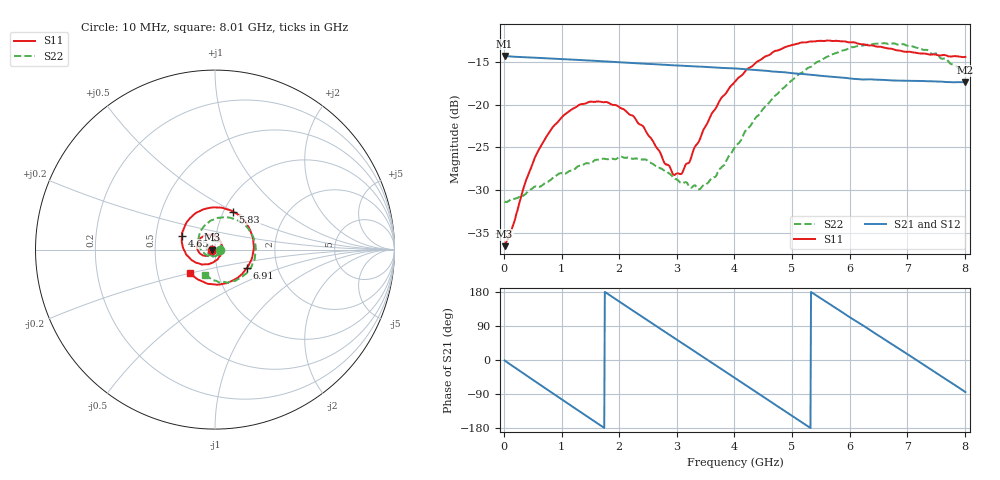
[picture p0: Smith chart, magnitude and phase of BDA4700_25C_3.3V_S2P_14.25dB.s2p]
!Agilent Technologies,E5071B,MY42404982,A.09.10
!Date: Mon Oct 20 18:09:01 2025
!Data & Calibration Information:
!Freq	S11:SOLT2(ON)	S21:SOLT2(ON)	S12:SOLT2(ON)	S22:SOLT2(ON)
# Hz S RI R 50
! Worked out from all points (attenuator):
!   801 points, 10 MHz to 8.01 GHz, reference 50 ohm
!   highest |S21| = -14.34 dB at 10 MHz (marker M1); lowest = -17.4 dB at 8 GHz (marker M2)
!   lowest |S11| = -36.5 dB at 10 MHz (marker M3), VSWR 1.03, Z = 48.5 - j0.125 ohm
!   |S11| at or under -10 dB: start of sweep to end of sweep
!   |S22| runs from -31.4 to -12.8 dB; largest |S21 - S12| = 0.0022
!   S11 on the Smith chart (normalised r, x): 10 MHz: 0.97, -0.00; 4.65 GHz: 0.68, +0.11; 5.83 GHz: 1.11, +0.50; 6.91 GHz: 1.39, -0.30; 8.01 GHz: 0.73, -0.19
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1e7  -0.0149 -0.00129  0.1917 -0.00424  0.1917 -0.00433  0.0271 -0.00099
6e8  -0.0417 -0.0347  0.0863 -0.166  0.0861 -0.166  0.0118 -0.031
1.01e9  -0.0815 -0.0238  -0.0467 -0.1781  -0.0466 -0.1781  -0.0196 -0.0347
1.35e9  -0.1002 0.0105  -0.1381 -0.1179  -0.1381 -0.1181  -0.0417 -0.0142
1.71e9  -0.087 0.0555  -0.1784 -0.012  -0.1785 -0.0118  -0.045 0.0174
2.07e9  -0.0458 0.0819  -0.148 0.095  -0.148 0.095  -0.0242 0.0427
2.41e9  0.00285 0.0748  -0.0675 0.1595  -0.0676 0.1596  0.007 0.0474
2.68e9  0.031 0.0447  0.0125 0.1708  0.0123 0.1708  0.0265 0.0336
2.94e9  0.0388 0.00447  0.0853 0.1464  0.0852 0.146  0.0352 0.0133
3.08e9  0.0347 -0.0185  0.1181 0.1201  0.1169 0.1209  0.0348 -0.00021
3.41e9  -0.000874 -0.064  0.1623 0.0365  0.1624 0.0365  0.0182 -0.0267
3.67e9  -0.0474 -0.0817  0.16 -0.0382  0.16 -0.0387  -0.00633 -0.0374
4.01e9  -0.1194 -0.065  0.1093 -0.1201  0.1094 -0.1199  -0.047 -0.031
4.65e9  -0.1838 0.0779  -0.0592 -0.1443  -0.0589 -0.1447  -0.092 0.0556
5.35e9  -0.0538 0.2271  -0.1487 0.00636  -0.1488 0.00554  -0.00544 0.1678
5.83e9  0.1003 0.2118  -0.0929 0.11  -0.0924 0.11  0.1158 0.1676
6.25e9  0.1956 0.11  0.00115 0.1399  0.00331 0.1398  0.2026 0.0893
6.68e9  0.2093 -0.0345  0.0945 0.1014  0.0948 0.1013  0.2238 -0.0294
6.91e9  0.1764 -0.1044  0.125 0.0574  0.1252 0.0567  0.2046 -0.0939
7.46e9  0.0187 -0.1952  0.1184 -0.0679  0.1184 -0.068  0.0791 -0.1809
8e9  -0.1381 -0.1298  0.0148 -0.134  0.0152 -0.1342  -0.0519 -0.1419
8.01e9  -0.1401 -0.1279  0.0125 -0.1343  0.013 -0.1343  -0.0537 -0.1399
